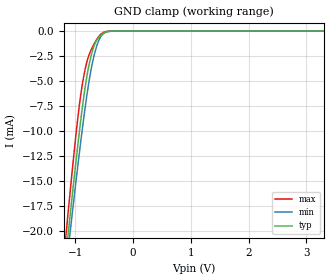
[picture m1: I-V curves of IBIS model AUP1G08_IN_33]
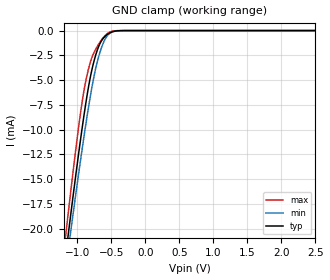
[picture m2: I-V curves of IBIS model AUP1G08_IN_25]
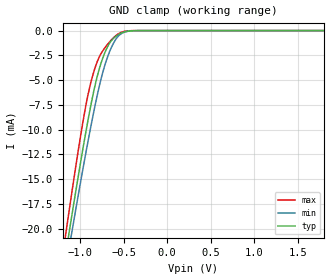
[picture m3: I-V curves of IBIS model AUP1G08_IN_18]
| TEXAS INSTRUMENTS INCORPORATED
| Standard Linear and Logic Group
| IBIS Model of SN74AUP1G08
| LOW POWER SINGLE 2-INPUT POSITIVE-AND GATE
| This file contains package information for the following:
|  SOT 5-pin (DCK) package as [Component] AUP1G08_DCK
|  SOT 5-pin (DBV) package as [Component] AUP1G08_DBV
|  NanoStar WCSP 5-pin (YEP) package as [Component] AUP1G08_YEP
|  NanoFree WCSP 5-pin (YZP) package as [Component] AUP1G08_YZP
| This device can be powered at the following Vccs:
|  3.3 volt Vcc
|  2.5 volt Vcc
|  1.8 volt Vcc
|  1.5 volt Vcc
|  1.2 volt Vcc
|  0.8 volt Vcc
| This file provides unique models under the [Model Selector] for each Vcc.
| For operation at a specific Vcc, select the appropriate model after each
| [Model Selector] keyword.
[IBIS Ver]   3.2
[Comment char]  |_char
[File Name]   sn74aup1g08.ibs
[File Rev]   1.2 | x_die
[Date]   08/30/04
[Source]   Data created from TI-SPICE simulations at TI-SLL.
[Notes]   The following is an IBIS list for the AUP1G08.
   Please contact sllibis@ti.com with questions and
   comments concerning SLL IBIS models.
   - FILE REV HISTORY
   - 1.1 Release IBIS file on 01/16/04
   - 1.2 YEP and YZP packages released on 08/27/04
   - Power clamp data deleted as there is no power-clamp diode.
   - Non-monotonic data in pullup data due to resistor at output.
[Disclaimer] Property of Texas Instruments Incorporated.  Unauthorized
   reproduction and/or distribution is strictly prohibited.
   This product is protected under copyright law.
   Created  2004, (C) Copyright  2004, Texas Instruments
   Incorporated, All Rights Reserved
   UNLESS THERE IS A SIGNED, WRITTEN AGREEMENT TO THE
   CONTRARY, TEXAS INSTRUMENTS (TI) IS PROVIDING THE IBIS
   MODELS  AND WITHOUT ANY WARRANTY, EXPRESSED OR
   IMPLIED.  TI assumes no liability for:
   1) the accuracy of the IBIS models provided to your
   company;
   2) the proper functioning of these IBIS Models in your
   design or for any resulting applications; or
   3) infringement of patents, copyrights or intellectual
   property rights resulting from your use of these IBIS
   models.
   TI provides IBIS Models as a service to our customers.
   You and your company shall not distribute, sell or give
   these models to anyone else without prior written
   permission from TI.
   TI reserves the right to make changes to our products or
   to discontinue any semiconductor product or service
   without notice, and advises our customers to obtain the
   latest version of relevant information to verify, before
   placing orders, that the information being relied on is
   current.
   Please be aware that your receipt and use of the IBIS
   information provided shall serve as acceptance of these
   terms and conditions.  If you do not accept these terms,
   you should return or destroy the IBIS models and any
   other accompanying information immediately.
| Component AUP1G08_DCK 5-pin SOT
[Component]   AUP1G08_DCK
[Manufacturer]   Texas Instruments, Inc.
[Package]
|   typ   min   max
R_pkg   2.000e-02   1.700e-02   2.500e-02
L_pkg   9.980e-10   8.810e-10   1.069e-09
C_pkg   1.460e-13   1.180e-13   2.050e-13
[Pin]   signal_name   model_name   R_pin   L_pin   C_pin
1   A   AUP1G08_IN   1.900e-02   1.069e-09   1.620e-13
2   B   AUP1G08_IN   1.800e-02   8.810e-10   1.210e-13
3   GND   GND   1.700e-02   1.031e-09   2.050e-13
4   Y   AUP1G08_OUT   2.000e-02   9.600e-10   1.240e-13
5   VCC   POWER   2.500e-02   1.049e-09   1.180e-13
| Component AUP1G08_DBV 5-pin SOT
[Component]   AUP1G08_DBV
[Manufacturer]   Texas Instruments, Inc.
[Package]
|   typ   min   max
R_pkg   2.500e-02   2.100e-02   2.900e-02
L_pkg   1.529e-09   1.312e-09   1.906e-09
C_pkg   1.560e-13   1.100e-13   2.400e-13
[Pin]   signal_name   model_name   R_pin   L_pin   C_pin
1   A   AUP1G08_IN   2.100e-02   1.511e-09   1.440e-13
2   B   AUP1G08_IN   2.300e-02   1.312e-09   1.380e-13
3   GND   GND   2.900e-02   1.906e-09   2.400e-13
4   Y   AUP1G08_OUT   2.600e-02   1.541e-09   1.500e-13
5   VCC   POWER   2.500e-02   1.374e-09   1.100e-13
| Component AUP1G08_YEP 5-pin NanoStar WCSP
[Component]   AUP1G08_YEP
[Manufacturer]   Texas Instruments, Inc.
[Package]
|   typ   min   max
R_pkg   0.001   0.001   0.001
L_pkg   0.021nH   0.021nH   0.021nH
C_pkg   0.046pF   0.045pF   0.047pF
[Pin]   signal_name   model_name   R_pin   L_pin   C_pin
1   A   AUP1G08_IN   0.001   0.021nH   0.046pF
2   B   AUP1G08_IN   0.001   0.021nH   0.047pF
3   GND   GND   0.001   0.021nH   0.046pF
4   Y   AUP1G08_OUT   0.001   0.021nH   0.045pF
5   VCC   POWER   0.001   0.021nH   0.045pF
| Component AUP1G08_YZP 5-pin NanoStar WCSP
[Component]   AUP1G08_YZP
[Manufacturer]   Texas Instruments, Inc.
[Package]
|   typ   min   max
R_pkg   0.001   0.001   0.001
L_pkg   0.021nH   0.021nH   0.021nH
C_pkg   0.046pF   0.045pF   0.047pF
[Pin]   signal_name   model_name   R_pin   L_pin   C_pin
1   A   AUP1G08_IN   0.001   0.021nH   0.046pF
2   B   AUP1G08_IN   0.001   0.021nH   0.047pF
3   GND   GND   0.001   0.021nH   0.046pF
4   Y   AUP1G08_OUT   0.001   0.021nH   0.045pF
5   VCC   POWER   0.001   0.021nH   0.045pF
| Model AUP1G08_IN
[Model Selector]   AUP1G08_IN
AUP1G08_IN_33   3.3 volt Vcc
AUP1G08_IN_25   2.5 volt Vcc
AUP1G08_IN_18   1.8 volt Vcc
AUP1G08_IN_15   1.5 volt Vcc
AUP1G08_IN_12   1.2 volt Vcc
AUP1G08_IN_08   0.8 volt Vcc
| Model AUP1G08_OUT
[Model Selector]   AUP1G08_OUT
AUP1G08_OUT_33   3.3 volt Vcc
AUP1G08_OUT_25   2.5 volt Vcc
AUP1G08_OUT_18   1.8 volt Vcc
AUP1G08_OUT_15   1.5 volt Vcc
AUP1G08_OUT_12   1.2 volt Vcc
AUP1G08_OUT_08   0.8 volt Vcc
| Models and submodels in the file (12): AUP1G08_IN_33 (Input), AUP1G08_IN_25 (Input), AUP1G08_IN_18 (Input), AUP1G08_IN_15 (Input), AUP1G08_IN_12 (Input), AUP1G08_IN_08 (Input), AUP1G08_OUT_33 (Output), AUP1G08_OUT_25 (Output), AUP1G08_OUT_18 (Output), AUP1G08_OUT_15 (Output), AUP1G08_OUT_12 (Output), AUP1G08_OUT_08 (Output)
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[Model]   AUP1G08_IN_33
Model_type  Input
Vinl=0.9
Vinh=2
| variable   typ   min   max
C_comp   1.41pF   1.15pF   1.78pF
[Temperature Range]   40   100   -40
| Ambient temperature   25   85   -40
[Voltage range]   3.3   3   3.6
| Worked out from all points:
|   GND clamp passes 1 mA (typ) near -0.64 V on its own axis
[GND Clamp]
| AUP1G08_IN_33
|   Voltage   I(typ)   I(min)   I(max)
-3.6V     -171.6mA   -163.5mA   -181.1mA
-1.16V    -22.22mA   -23.69mA   -20.18mA
-1.11V    -19.45mA   -21.09mA   -17.19mA
-1.085V   -18.08mA   -19.81mA   -15.71mA
-940mV    -10.5mA    -12.6mA    -7.822mA
-890mV    -8.117mA   -10.26mA   -5.698mA
-835mV    -5.768mA   -7.825mA   -3.925mA
-755mV    -3.153mA   -4.717mA   -2.255mA
-675mV    -1.463mA   -2.419mA   -1.277mA
-595mV    -617.7uA   -945.8uA   -546.7uA
-515mV    -215.4uA   -248.8uA   -134.4uA
3.3V      132.2pA    540.4pA    36.28pA
[Model]   AUP1G08_IN_25
Model_type  Input
Vinl=0.7
Vinh=1.6
| variable   typ   min   max
C_comp   1.44pF   1.20pF   1.77pF
[Temperature Range]   40   100   -40
| Ambient temperature   25   85   -40
[Voltage range]   2.5   2.3   2.7
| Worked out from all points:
|   GND clamp passes 1 mA (typ) near -0.64 V on its own axis
[GND Clamp]
| AUP1G08_IN_25
|   Voltage   I(typ)   I(min)   I(max)
-3.6V     -171.6mA   -163.5mA   -181.1mA
-1.165V   -22.5mA    -23.95mA   -20.48mA
-1.115V   -19.72mA   -21.35mA   -17.49mA
-1.09V    -18.36mA   -20.06mA   -16.01mA
-945mV    -10.75mA   -12.84mA   -8.061mA
-890mV    -8.117mA   -10.26mA   -5.698mA
-835mV    -5.768mA   -7.825mA   -3.925mA
-760mV    -3.287mA   -4.89mA    -2.329mA
-675mV    -1.463mA   -2.419mA   -1.277mA
-595mV    -617.7uA   -945.8uA   -546.7uA
-520mV    -233.1uA   -272.6uA   -149.9uA
2.5V      104.3pA    491.9pA    26.71pA
[Model]   AUP1G08_IN_18
Model_type  Input
Vinl=0.6825
Vinh=1.0725
| variable   typ   min   max
C_comp   1.49pF   1.27pF   1.76pF
[Temperature Range]   40   100   -40
| Ambient temperature   25   85   -40
[Voltage range]   1.8   1.65   1.95
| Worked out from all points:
|   GND clamp passes 1 mA (typ) near -0.64 V on its own axis
[GND Clamp]
| AUP1G08_IN_18
|   Voltage   I(typ)   I(min)   I(max)
-3.6V     -171.6mA   -163.5mA   -181.1mA
-1.16V    -22.22mA   -23.69mA   -20.18mA
-1.135V   -20.83mA   -22.39mA   -18.68mA
-1.11V    -19.45mA   -21.09mA   -17.19mA
-1.09V    -18.36mA   -20.06mA   -16.01mA
-960mV    -11.5mA    -13.57mA   -8.799mA
-850mV    -6.372mA   -8.471mA   -4.359mA
-780mV    -3.86mA    -5.615mA   -2.659mA
-710mV    -2.096mA   -3.313mA   -1.67mA
-625mV    -855.5uA   -1.409mA   -788.9uA
-540mV    -313.2uA   -390uA     -224.9uA
1.8V      83.14pA    451.3pA    18.98pA
